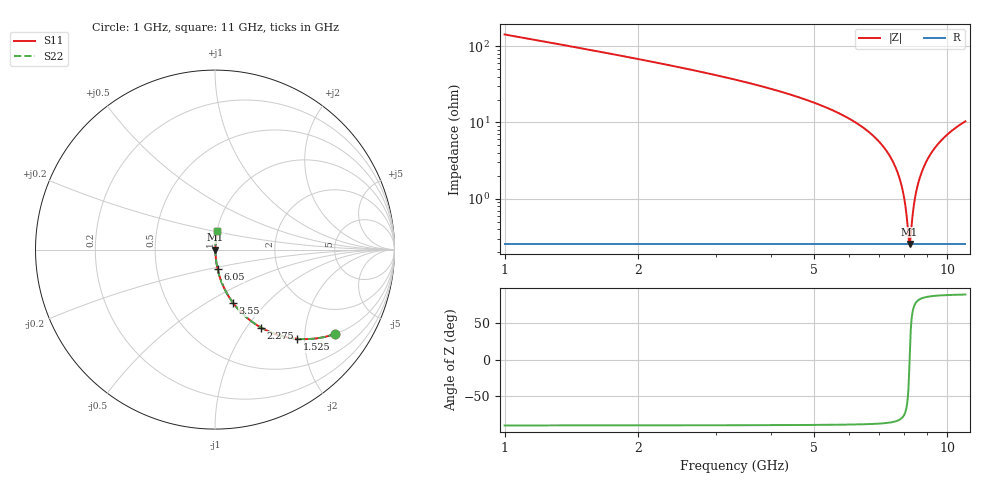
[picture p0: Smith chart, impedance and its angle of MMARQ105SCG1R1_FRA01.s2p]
! MMARQ105SCG1R1_FRA01  S-PARAMETER MODEL  ( General Type )
! Model Generated by TAIYO YUDEN Corporation (http://www.ty-top.com)
! Version 1.0
! TAIYO YUDEN Control No. 200326
! Copyright(c) 2020 TAIYO YUDEN CO.,LTD. All Rights Reserved.
! Product Description (link to TY-COMPAS)
! https://ds.yuden.co.jp/TYCOMPAS/or/detail?pn=MMARQ105SCG1R1BFRA01&u=M
! Products Name : Multilayer Ceramic Capacitors
! Characteristics :
!  Capacitance : 1.1 pF , Rated Voltage : 250V , TCC : CG / C0G
!  Case Size : 1.0 x 0.5 / 0.039 x 0.02 [mm/inch] , Thickness : 0.5 / 0.02 [mm/inch]
!  (Conditions: Temperature = 25 degC , DC Bias Current/Voltage = 0A / 0V)
! External Node Assignments :
!  1  o---| |---o  2
! GND o---------o GND
! Frequency Range : 1GHz  -  11GHz  [ 401 STEP ]
# MHz S RI R 50
! Freq[MHz].  S11 Real  S11 Imag  S21 Real  S21 Imag  S12 Real  S12 Imag  S22 Real  S22 Imag
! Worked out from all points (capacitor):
!   401 points, 1 GHz to 11 GHz, reference 50 ohm
!   read as one part in series: C = 1.1 pF near 1.05 GHz
!   lowest |Z| = 256 mohm at 8.225 GHz (marker M1)
!   series resonance near 8.227 GHz, so ESL is about 340 pH
!   S11 on the Smith chart (normalised r, x): 1 GHz: 1.01, -2.85; 1.525 GHz: 1.01, -1.83; 2.275 GHz: 1.01, -1.17; 3.55 GHz: 1.01, -0.66; 6.05 GHz: 1.01, -0.22; 11 GHz: 1.01, +0.21
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1000  0.6697 -0.4694  0.3303 0.4694  0.3303 0.4694  0.6697 -0.4694
1525  0.4562 -0.4967  0.5438 0.4967  0.5438 0.4967  0.4562 -0.4967
2275  0.2572 -0.4349  0.7428 0.4349  0.7428 0.4349  0.2572 -0.4349
2675  0.1907 -0.3902  0.8093 0.3902  0.8093 0.3902  0.1907 -0.3902
3550  0.1009 -0.2973  0.8991 0.2973  0.8991 0.2973  0.1009 -0.2973
4350  0.0564 -0.2254  0.9436 0.2254  0.9436 0.2254  0.0564 -0.2254
6000  0.015 -0.1108  0.985 0.1108  0.985 0.1108  0.015 -0.1108
6050  0.0144 -0.1079  0.9856 0.1079  0.9856 0.1079  0.0144 -0.1079
7050  0.00549 -0.0541  0.9945 0.0541  0.9945 0.0541  0.00549 -0.0541
7675  0.00315 -0.0243  0.9969 0.0243  0.9969 0.0243  0.00315 -0.0243
7975  0.00267 -0.0109  0.9973 0.0109  0.9973 0.0109  0.00267 -0.0109
8075  0.0026 -0.00654  0.9974 0.00654  0.9974 0.00654  0.0026 -0.00654
8175  0.00256 -0.00223  0.9974 0.00223  0.9974 0.00223  0.00256 -0.00223
8225  0.00255 -9.86e-05  0.9974 9.86e-05  0.9974 9.86e-05  0.00255 -9.86e-05
8275  0.00256 0.00202  0.9974 -0.00202  0.9974 -0.00202  0.00256 0.00202
8375  0.00259 0.00622  0.9974 -0.00622  0.9974 -0.00622  0.00259 0.00622
8450  0.00264 0.00934  0.9974 -0.00934  0.9974 -0.00934  0.00264 0.00934
8625  0.00283 0.0165  0.9972 -0.0165  0.9972 -0.0165  0.00283 0.0165
8925  0.00337 0.0285  0.9966 -0.0285  0.9966 -0.0285  0.00337 0.0285
9350  0.00457 0.0448  0.9954 -0.0448  0.9954 -0.0448  0.00457 0.0448
10050  0.0075 0.0701  0.9925 -0.0701  0.9925 -0.0701  0.0075 0.0701
11000  0.0131 0.1019  0.9869 -0.1019  0.9869 -0.1019  0.0131 0.1019
